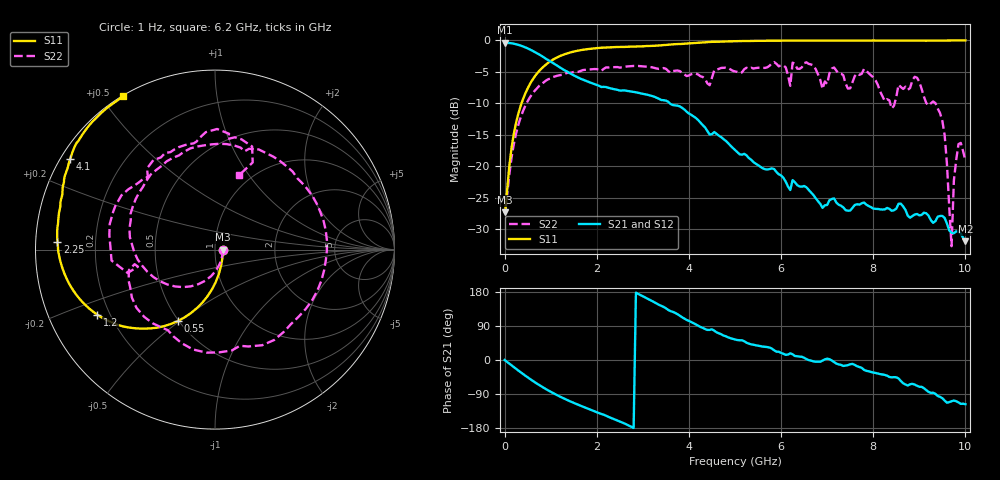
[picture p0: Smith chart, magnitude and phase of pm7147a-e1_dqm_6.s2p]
# GHz S DB R 50
! S-Parameters data
! Freq  dbS11  angS11  dbS21  angS21  dbS12  angS12  dbS22  angS22
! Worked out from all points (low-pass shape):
!   279 points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, 1 Hz to 10 GHz, reference 50 ohm
!   highest |S21| = -0.38 dB at 25.12 kHz (marker M1); lowest = -32.0 dB at 10 GHz (marker M2)
!   |S21| within 3 dB of the highest: start of sweep to 997.4 MHz
!   lowest |S11| = -27.3 dB at 25.12 kHz (marker M3), VSWR 1.09, Z = 54.5 - j0.00234 ohm
!   |S11| at or under -10 dB: start of sweep to 368.3 MHz
!   |S22| runs from -32.7 to -3.5 dB; largest |S21 - S12| = 0
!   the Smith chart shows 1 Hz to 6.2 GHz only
!   S11 on the Smith chart (normalised r, x): 1 Hz: 1.09, -0.00; 550 MHz: 0.49, -0.49; 1.2 GHz: 0.15, -0.25; 2.25 GHz: 0.06, +0.02; 4.1 GHz: 0.03, +0.29; 6.2 GHz: 0.00, +0.57
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1e-09  -27.34 -0.0  -0.38 -0.0  -0.38 -0.0  -27.34 -0.0
2.51189e-05  -27.34 -0.0  -0.38 -0.0  -0.38 -0.0  -27.34 -0.0
0.2  -14.87 -88.6  -0.53 -18.8  -0.53 -18.8  -16.51 -98.3
0.55  -6.95 -117.6  -1.45 -50.0  -1.45 -50.0  -9.05 -149.8
1.2  -2.50 -151.1  -4.30 -96.5  -4.30 -96.5  -5.54 143.0
1.7  -1.50 -168.7  -6.24 -123.1  -6.24 -123.1  -4.72 103.6
2.25  -1.12 177.2  -7.54 -149.9  -7.54 -149.9  -4.32 61.8
2.9  -0.97 165.1  -8.35 174.5  -8.35 174.5  -4.07 4.7
3.35  -0.81 158.7  -9.29 145.6  -9.29 145.6  -4.54 -44.3
4.1  -0.43 148.1  -12.09 97.2  -12.09 97.2  -5.29 -136.5
5.05  -0.12 134.7  -17.78 52.6  -17.78 52.6  -5.02 135.1
5.85  -0.07 124.9  -20.48 25.7  -20.48 25.7  -3.45 89.0
6.2  -0.04 121.0  -23.81 17.5  -23.81 17.5  -7.23 72.1
6.7  -0.03 115.8  -24.59 -3.6  -24.59 -3.6  -3.98 43.3
8.35  -0.02 101.2  -26.81 -44.8  -26.81 -44.8  -9.54 -15.8
8.85  -0.04 97.4  -27.95 -62.9  -27.95 -62.9  -6.32 -25.3
9.45  -0.03 93.4  -27.94 -97.3  -27.94 -97.3  -11.57 -109.5
9.55  -0.03 92.7  -28.25 -107.0  -28.25 -107.0  -15.08 -153.1
9.7  -0.02 91.7  -30.63 -108.8  -30.63 -108.8  -32.74 13.2
9.75  -0.02 91.3  -30.68 -106.9  -30.68 -106.9  -22.31 -40.8
9.85  -0.02 90.7  -30.44 -112.0  -30.44 -112.0  -16.51 -70.1
10  -0.02 89.7  -31.99 -116.8  -31.99 -116.8  -19.15 -130.7
